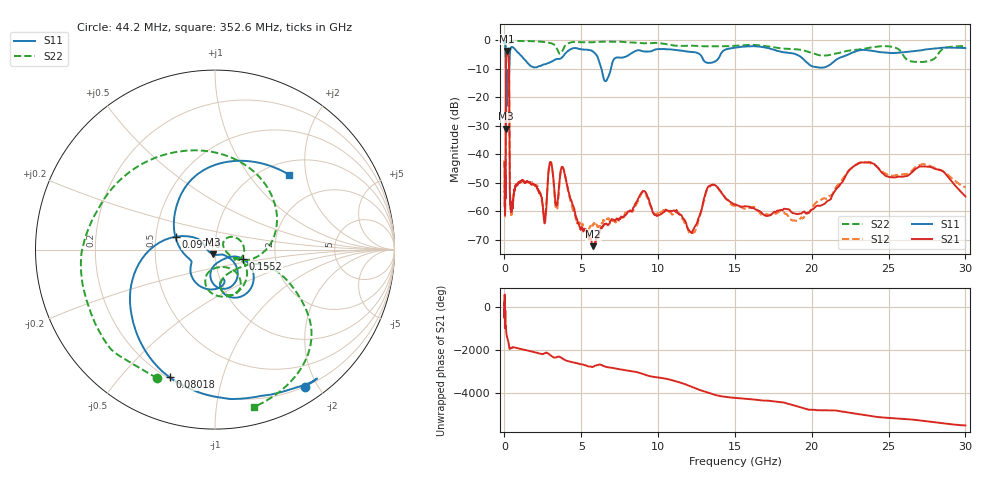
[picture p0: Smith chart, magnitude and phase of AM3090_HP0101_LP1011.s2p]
! Date/Time: Thu, Feb 28, 2019 1:59 PM
! Network Analyzer: Agilent Technologies E8364B Rev: A.07.50.67
! Sweep from 0.010 to 30.000 GHz, 1601 Points, Sweep Type: LOG
! Power Supply: 5.023 V, 0.002 A
# Hz S DB R 50
!freq MagS11 AngS11 MagS21 AngS21 MagS12 AngS12 MagS22 AngS22
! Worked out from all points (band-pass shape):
!   1601 points, 10 MHz to 30 GHz, reference 50 ohm
!   highest |S21| = -3.85 dB at 157.6 MHz (marker M1); lowest = -72.3 dB at 5.783 GHz (marker M2)
!   |S21| within 3 dB of the highest: 108.3 MHz to 284.8 MHz (176.5 MHz wide, 89.8 % of centre)
!   lowest |S11| = -31.1 dB at 105.1 MHz (marker M3), VSWR 1.06, Z = 48.9 - j2.55 ohm
!   |S11| at or under -10 dB: 95.92 MHz to 314.3 MHz (218.4 MHz wide, 106 % of centre); 6.308 GHz to 6.931 GHz (622.2 MHz wide, 9.4 % of centre)
!   |S22| runs from -26.1 to -0.1 dB; largest |S21 - S12| = 0.013
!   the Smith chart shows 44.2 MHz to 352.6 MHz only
!   S11 on the Smith chart (normalised r, x): 44.2 MHz: 0.19, -1.83; 80.18 MHz: 0.21, -0.68; 97.46 MHz: 0.64, +0.10; 155.2 MHz: 1.36, -0.14; 352.6 MHz: 1.26, +1.60
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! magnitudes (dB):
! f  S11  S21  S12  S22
! 10 MHz  -0.3  -43.0  -45.0  -0.7
! 38.04 MHz  -0.5  -60.7  -59.4  -1.7
! 44.2 MHz  -0.8  -57.3  -56.4  -2.1
! 80.18 MHz  -2.4  -52.4  -48.9  -4.6
! 97.46 MHz  -12.9  -15.3  -15.3  -12.4
! 105.1 MHz  -31.1  -8.0  -8.0  -25.5
! 120.9 MHz  -13.1  -5.1  -5.1  -16.8
! 144.7 MHz  -23.0  -4.0  -4.0  -18.4
! 155.2 MHz  -15.8  -3.9  -3.8  -16.4
! 157.6 MHz  -14.5  -3.8  -3.8  -15.7
! 288.7 MHz  -15.8  -7.4  -7.4  -15.5
! 352.6 MHz  -4.6  -53.4  -51.8  -0.9
! 550.5 MHz  -2.6  -57.6  -56.8  -0.3
! 2.084 GHz  -9.6  -51.5  -51.0  -0.5
! 2.623 GHz  -8.5  -64.1  -61.8  -0.7
! 2.958 GHz  -7.8  -43.1  -43.1  -1.0
! 3.385 GHz  -6.7  -58.1  -59.5  -2.7
! 3.798 GHz  -5.8  -44.7  -44.7  -3.5
! 5.783 GHz  -4.1  -72.3  -64.8  -0.7
! 7.926 GHz  -5.8  -61.1  -60.4  -0.7
! 23.36 GHz  -3.4  -43.0  -42.9  -3.1
! 30 GHz  -2.8  -54.8  -51.7  -2.1
